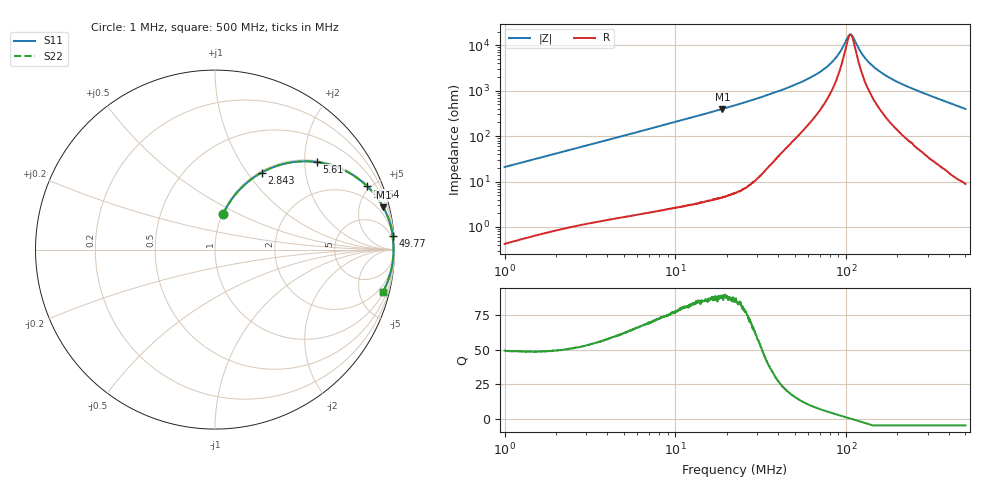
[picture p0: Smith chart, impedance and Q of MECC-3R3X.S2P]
!s-Parameter Generated by FASTRON Sdn. Bhd.
!FASTRON P/N : MECC-3R3X
!Keysight Technologies,E4991B,MY54100416,A.01.15
!Date: Mon Mar 16 14:57:02 2026
!Version  : Rev00 Mon Mar 16 14:57:02 2026
!Data & Calibration Information:
!PortZ  Port1:50+j0  Port2:50+j0
!When reading, reference impedance value at option line is always used.
!Remarks : This data is being provided solely for informational purposes.
!Freq	S11	S21	S12	S22
# Hz S dB R 50
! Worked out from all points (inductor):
!   1601 points, 1 MHz to 500 MHz, reference 50 ohm
!   read as one part in series: L = 3.31 uH near 1.032 MHz
!   highest Q = 89.1 at 18.85 MHz (marker M1), where L = 3.35 uH
!   self-resonance near 105.7 MHz
!   S11 on the Smith chart (normalised r, x): 1 MHz: 1.01, +0.42; 2.843 MHz: 1.02, +1.17; 5.61 MHz: 1.04, +2.30; 11.64 MHz: 1.06, +4.79; 49.77 MHz: 3, +27; 500 MHz: 1.18, -7.95
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1000000  -13.83 77.1  -0.22 -11.7  -0.22 -11.7  -13.83 77.1
1749473  -9.41 69.0  -0.59 -19.8  -0.59 -19.8  -9.41 69.0
2820919  -6.05 59.0  -1.33 -29.9  -1.33 -29.9  -6.05 59.0
2842918  -6.00 58.9  -1.35 -30.1  -1.35 -30.1  -6.00 58.9
5610017  -2.52 40.7  -3.72 -48.5  -3.72 -48.5  -2.52 40.7
7957584  -1.44 31.3  -5.69 -57.9  -5.69 -57.9  -1.44 31.3
1.164376e7  -0.73 22.5  -8.33 -66.8  -8.33 -66.8  -0.73 22.5
1.884792e7  -0.29 14.1  -12.26 -75.2  -12.26 -75.2  -0.29 14.1
2.236068e7  -0.21 11.8  -13.79 -77.5  -13.79 -77.5  -0.21 11.8
4.977112e7  -0.06 4.3  -22.56 -82.1  -22.56 -82.1  -0.06 4.3
6.307767e7  -0.06 2.8  -26.19 -81.0  -26.19 -81.0  -0.06 2.8
7.425464e7  -0.05 1.9  -29.57 -78.4  -29.57 -78.4  -0.05 1.9
8.408199e7  -0.05 1.2  -33.20 -73.7  -33.20 -73.7  -0.05 1.2
9.229699e7  -0.05 0.7  -37.17 -64.9  -37.17 -64.9  -0.05 0.7
1.025021e8  -0.05 0.2  -43.74 -28.5  -43.74 -28.5  -0.05 0.2
1.061486e8  -0.05 -0.0  -44.79 0.4  -44.79 0.4  -0.05 -0.0
1.099249e8  -0.05 -0.2  -43.66 28.9  -43.66 28.9  -0.05 -0.2
1.216058e8  -0.05 -0.7  -37.28 64.9  -37.28 64.9  -0.05 -0.7
1.340065e8  -0.05 -1.2  -33.08 74.1  -33.08 74.1  -0.05 -1.2
1.77937e8  -0.06 -2.9  -25.97 80.8  -25.97 80.8  -0.06 -2.9
2.623928e8  -0.09 -5.7  -20.08 81.3  -20.08 81.3  -0.09 -5.7
5e8  -0.31 -14.0  -12.30 74.7  -12.30 74.7  -0.31 -14.0
